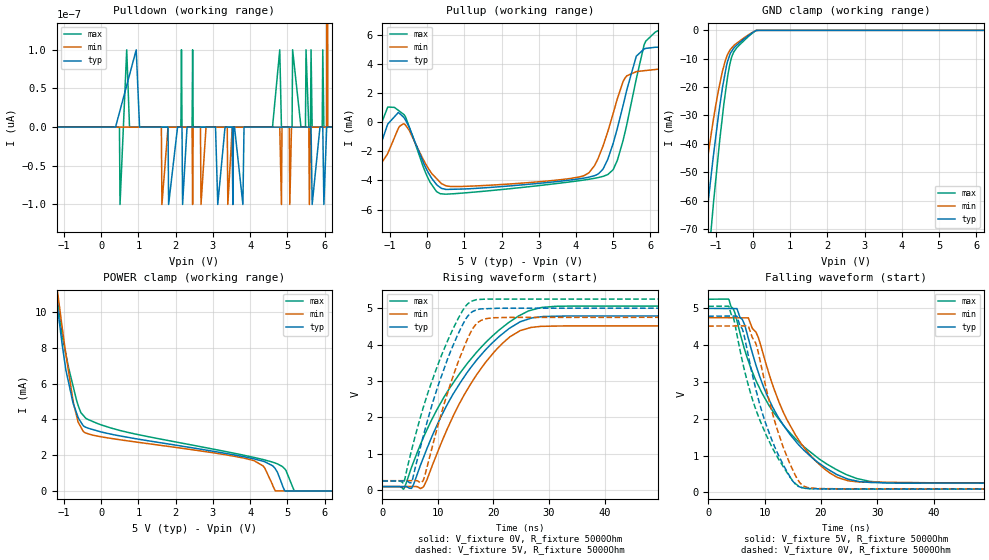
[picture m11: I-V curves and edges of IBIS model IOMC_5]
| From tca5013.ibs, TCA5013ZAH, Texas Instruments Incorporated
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[Model]   IOMC_5
Model_type   I/O
Polarity   Non-Inverting
Enable   Active-Low
Vinl = 1.5
Vinh = 3.5
Vmeas = 2.5
Vref = 5
Cref = 1pF
Rref = 5000
|   typ   min   max
C_comp   0.937p   0.723p   1.081p
|C_comp (ON state)   0.950p   0.730p   1.090p
|C_comp (OFF state)   0.937p   0.723p   1.081p
[Model spec]
|subparameter
Vinl   1.5   1.425   1.575
Vinh   3.5   3.325   3.675
[Voltage Range]   5   4.75   5.25
[Temperature Range]   27   125   -40
[Pullup Reference]   5   4.75   5.25
[Pulldown Reference]   0   0   0
[Power Clamp Reference]   5   4.75   5.25
[GND Clamp Reference]   0   0   0
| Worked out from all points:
|   slope of the pullup table from 0 to 0.75 V, typ, clamps not added: 577 ohm
|   GND clamp passes 1 mA (typ) near -0.03 V on its own axis
|   falling waveform, V_fixture 5V, R_fixture 5000Ohm: 20-80 % time 9.3ns typ, 7.76ns min, 11.1ns max; typ from 5 V to 0.246 V
|   rising waveform, V_fixture 0V, R_fixture 5000Ohm: 20-80 % time 10.8ns typ, 9.48ns min, 12.2ns max; typ from 0.089 V to 4.79 V
|   rising waveform, V_fixture 5V, R_fixture 5000Ohm: 20-80 % time 6.04ns typ, 5.57ns min, 6.66ns max; typ from 0.246 V to 5 V
|   falling waveform, V_fixture 0V, R_fixture 5000Ohm: 20-80 % time 5.48ns typ, 4.84ns min, 6.45ns max; typ from 4.79 V to 0.089 V
[Pulldown]
|   Voltage   I(typ)   I(min)   I(max)
-5V       0A         0A         0A
5.59V     0A         -100fA     0A
6.07V     0A         1pA        0A
6.805V    0A         -1pA       0A
6.82V     0A         0A         0A
7.48V     0A         -1pA       0A
7.495V    0A         0A         0A
8.65V     0A         0A         0A
8.665V    0A         0A         1pA
8.68V     0A         0A         0A
8.905V    0A         0A         1pA
10V       0A         0A         0A
[GND Clamp]
|   Voltage   I(typ)   I(min)   I(max)
-5V       -2.369A    -1.941A    -2.673A
-2.42V    -219.7mA   -176.2mA   -262.4mA
-1.25V    -66.28mA   -48.1mA    -89.27mA
-1.085V   -47mA      -33.52mA   -64.86mA
-905mV    -28.12mA   -19.9mA    -40.65mA
-815mV    -20.05mA   -14.29mA   -30.07mA
-680mV    -10.97mA   -8.543mA   -16.5mA
-605mV    -8.087mA   -6.745mA   -11.2mA
-515mV    -6.341mA   -5.437mA   -7.665mA
-365mV    -4.434mA   -3.879mA   -5.218mA
85mV      -45.91uA   -55.37uA   -59.48uA
10V       0A         0A         0A
[Pullup]
|   Voltage   I(typ)   I(min)   I(max)
-5V       -18.52mA   -15.06mA   -22.77mA
-1.88V    -4.765mA   -4.059mA   -5.417mA
-1.055V   -132.9uA   -2.139mA   1.036mA
-605mV    253.8uA    -141.3uA   465.6uA
355mV     -4.485mA   -4.136mA   -4.911mA
4.195V    -3.847mA   -3.688mA   -3.977mA
4.855V    -2.541mA   -642uA     -3.593mA
5.62V     4.524mA    3.461mA    2.976mA
6.295V    5.135mA    3.668mA    6.367mA
7.66V     4.946mA    4.221mA    6.395mA
8.065V    608.3uA    1.304mA    556uA
10V       72.03uA    88.68uA    71.46uA
[POWER Clamp]
|   Voltage   I(typ)   I(min)   I(max)
-5V       91.03mA    94.54mA    101.6mA
-1.25V    11.52mA    12.39mA    12.16mA
-1.055V   8.294mA    9.26mA     8.757mA
-755mV    4.909mA    5.036mA    5.866mA
-620mV    4.116mA    3.849mA    4.79mA
-425mV    3.572mA    3.247mA    4.094mA
4.09V     1.8mA      1.703mA    1.881mA
4.39V     1.633mA    1.289mA    1.734mA
4.66V     1.285mA    65.53uA    1.57mA
4.93V     0A         0A         1.237mA
5.185V    0A         0A         0A
10V       0A         0A         0A
[Ramp]
R_load = 5000
|   typ   min   max
dV/dt_r   2.82006/1.0795e-08   2.65774/9.45945e-09   2.98026/1.22453e-08
dV/dt_f   2.85232/9.2946e-09   2.69771/7.74469e-09   3.00156/1.11295e-08
[Falling Waveform]
V_fixture = 5V
V_fixture_min = 4.75V
V_fixture_max = 5.25V
R_fixture = 5000Ohm
C_fixture = 0F
|   Time   V(typ)   V(min)   V(max)
0s        5V         4.75V      5.25V
3.685ns   4.997V     4.746V     5.241V
5.096ns   4.996V     4.745V     4.663V
7.118ns   4.189V     4.743V     3.573V
8.874ns   3.27V      4.218V     2.91V
11.42ns   2.322V     2.927V     2.218V
16.51ns   1.221V     1.321V     1.307V
21.62ns   594.7mV    524.4mV    720.1mV
26.36ns   310.2mV    290.7mV    378.1mV
99.9ns    246mV      253.6mV    247.3mV
[Rising Waveform]
V_fixture = 0V
V_fixture_min = 0V
V_fixture_max = 0V
R_fixture = 5000Ohm
C_fixture = 0F
|   Time   V(typ)   V(min)   V(max)
0s        88.91mV    90.74mV    90.01mV
3.842ns   89.36mV    90.87mV    24.24mV
5.3ns     50.86mV    90.93mV    640.7mV
7.352ns   871.3mV    74.97mV    1.426V
11.58ns   2.32V      1.637V     2.669V
17ns      3.578V     3.176V     3.793V
21.62ns   4.293V     4.031V     4.47V
26.36ns   4.704V     4.452V     4.928V
33.52ns   4.784V     4.511V     5.056V
99.9ns    4.789V     4.52V      5.057V
[Rising Waveform]
V_fixture = 5V
V_fixture_min = 4.75V
V_fixture_max = 5.25V
R_fixture = 5000Ohm
C_fixture = 0F
|   Time   V(typ)   V(min)   V(max)
0s        246mV      253.5mV    247.4mV
3.842ns   246.6mV    253.7mV    188.1mV
5.3ns     228.2mV    253.8mV    1.117V
7.285ns   1.432V     241.9mV    2.224V
11.87ns   3.652V     2.73V      4.147V
14.42ns   4.532V     3.817V     4.925V
16.05ns   4.885V     4.376V     5.192V
17.78ns   4.98V      4.664V     5.242V
20.05ns   4.993V     4.736V     5.251V
99.9ns    5V         4.75V      5.25V
[Falling Waveform]
|Gnd
V_fixture = 0V
V_fixture_min = 0V
V_fixture_max = 0V
R_fixture = 5000Ohm
C_fixture = 0F
|   Time   V(typ)   V(min)   V(max)
0s        4.789V     4.52V      5.057V
3.685ns   4.792V     4.522V     5.049V
5.122ns   4.78V      4.523V     4.272V
6.215ns   4.364V     4.524V     3.463V
7.152ns   3.691V     4.507V     2.897V
8.63ns    2.693V     3.962V     2.178V
11.74ns   1.257V     1.969V     1.109V
14.46ns   437mV      792.2mV    429.1mV
16.96ns   118.5mV    173.2mV    117.7mV
99.9ns    88.91mV    90.74mV    90mV
